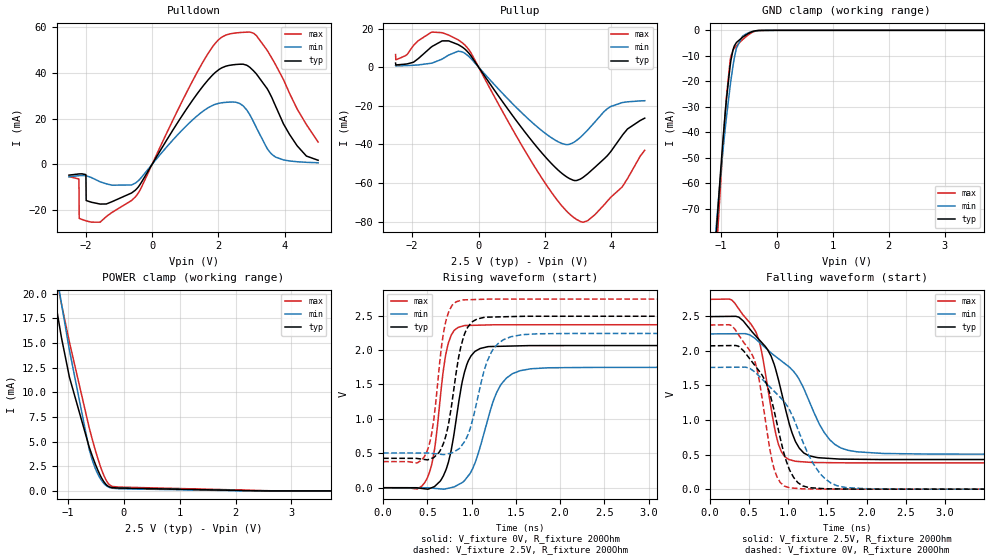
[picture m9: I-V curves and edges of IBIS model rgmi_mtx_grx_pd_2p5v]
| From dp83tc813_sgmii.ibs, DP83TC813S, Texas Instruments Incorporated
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| rgmi_mtx_grx_pd_2p5v
[Model]   rgmi_mtx_grx_pd_2p5v
Model_type   I/O
Polarity   Non-Inverting
Enable   Active-Low
Vinl = 0.7
Vinh = 1.7
Vmeas = 1.25
Vref = 1.25
Cref = 2pF
Rref = 100000
|   typ   min   max
C_comp   1.78pF   1.74pF   1.8pF
[Voltage Range]   2.5   2.25   2.75
[Temperature Range]   27   150   -40
[Pullup Reference]   2.5   2.25   2.75
[Pulldown Reference]   0   0   0
[Power Clamp Reference]   2.5   2.25   2.75
[GND Clamp Reference]   0   0   0
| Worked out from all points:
|   slope of the pulldown table from 0 to 0.375 V, typ, clamps not added: 41.3 ohm
|   slope of the pullup table from 0 to 0.375 V, typ, clamps not added: 39.8 ohm
|   GND clamp passes 1 mA (typ) near -0.49 V on its own axis
|   POWER clamp passes 1 mA (typ) near -0.36 V on its own axis
|   falling waveform, V_fixture 2.5V, R_fixture 200Ohm: 20-80 % time 347ps typ, 578ps min, 245ps max; typ from 2.49 V to 0.427 V
|   rising waveform, V_fixture 0V, R_fixture 200Ohm: 20-80 % time 169ps typ, 257ps min, 133ps max; typ from 0 V to 2.07 V
|   rising waveform, V_fixture 2.5V, R_fixture 200Ohm: 20-80 % time 160ps typ, 215ps min, 129ps max; typ from 0.427 V to 2.49 V
|   falling waveform, V_fixture 0V, R_fixture 200Ohm: 20-80 % time 311ps typ, 501ps min, 225ps max; typ from 2.07 V to 0 V
[Pulldown]
|   Voltage   I(typ)   I(min)   I(max)
-2.5V     -4.672mA   -5.389mA   -5.307mA
-2.208V   -4.173mA   -4.935mA   -6.345mA
-2.2V     -4.164mA   -4.928mA   -6.817mA
-2.192V   -4.156mA   -4.921mA   -23.54mA
-2.118V   -4.109mA   -4.872mA   -23.98mA
-1.99V    -4.622mA   -4.94mA    -24.62mA
-1.982V   -15.77mA   -4.953mA   -24.65mA
-617.5mV  -12.48mA   -8.98mA    -15.76mA
1.587V    35.18mA    23.8mA     46.1mA
2.428V    43.51mA    27.27mA    57.25mA
3.147V    39.41mA    15.86mA    56.18mA
5V        1.822mA    727.1uA    9.773mA
[GND Clamp]
|   Voltage   I(typ)   I(min)   I(max)
-2.5V     -599.2mA   -518.7mA   -673.8mA
-1.097V   -84.65mA   -80.59mA   -94.55mA
-1.045V   -67.67mA   -66.8mA    -74.76mA
-925mV    -32.91mA   -39.02mA   -33.16mA
-902.5mV  -27.45mA   -34.46mA   -26.56mA
-835mV    -13.97mA   -21.96mA   -11.93mA
-782.5mV  -7.567mA   -13.77mA   -7.699mA
-722.5mV  -4.782mA   -7.003mA   -6.022mA
-617.5mV  -2.807mA   -2.423mA   -3.769mA
-520mV    -1.387mA   -1.103mA   -1.953mA
-287.5mV  -43.21uA   -49.05uA   -52.55uA
5V        0A         0A         0A
[Pullup]
|   Voltage   I(typ)   I(min)   I(max)
-2.5V     2.111mA    768.5uA    6.54mA
-2.2V     1.575mA    804.7uA    5.936mA
-1.96V    2.572mA    997.9uA    11.28mA
-1.39V    10.84mA    2.186mA    18.18mA
-902.5mV  13.62mA    6.256mA    16.65mA
-467.5mV  10.11mA    7.704mA    12.3mA
2.083V    -47.91mA   -35.26mA   -62.11mA
2.638V    -56.7mA    -40.12mA   -74.4mA
3.065V    -57.97mA   -36.33mA   -79.98mA
3.973V    -43.87mA   -20.44mA   -67.55mA
4.482V    -32.02mA   -17.96mA   -57.74mA
5V        -26.43mA   -17.39mA   -43.06mA
[POWER Clamp]
|   Voltage   I(typ)   I(min)   I(max)
-2.5V     127.6mA    94.09mA    171.5mA
-1.232V   19.61mA    23.09mA    22.45mA
-1.113V   15.56mA    19mA       18.96mA
-970mV    11.54mA    14.28mA    15.09mA
-617.5mV  4.476mA    4.246mA    6.44mA
-550mV    3.38mA     2.956mA    5.003mA
-460mV    2.088mA    1.696mA    3.259mA
-355mV    942.8uA    770.4uA    1.589mA
-272.5mV  461.3uA    397.3uA    740.3uA
-197.5mV  326.8uA    269.2uA    451.3uA
-25mV     285.4uA    216.3uA    382.5uA
5V        0A         0A         0A
[Ramp]
R_load = 200
|   typ   min   max
dV/dt_r   1.24108/1.68325e-10   1.05398/2.5536e-10   1.42125/1.32406e-10
dV/dt_f   1.23796/3.45009e-10   1.04176/5.77786e-10   1.41626/2.44193e-10
[Falling Waveform]
V_fixture = 2.5V
V_fixture_min = 2.25V
V_fixture_max = 2.75V
R_fixture = 200Ohm
C_fixture = 0F
|   Time   V(typ)   V(min)   V(max)
0s        2.491V     2.241V     2.74V
280.5ps   2.494V     2.243V     2.731V
578.4ps   2.223V     2.176V     2.291V
660.5ps   2.121V     2.092V     1.991V
873.9ps   1.591V     1.886V     658.7mV
1.083ns   716.5mV    1.681V     405.7mV
1.201ns   521.6mV    1.45V      393.8mV
1.529ns   443.4mV    715.6mV    382.4mV
1.881ns   431.5mV    539mV      379.9mV
12ns      427.3mV    504.7mV    379.4mV
[Rising Waveform]
V_fixture = 0V
V_fixture_min = 0V
V_fixture_max = 0V
R_fixture = 200Ohm
C_fixture = 0F
|   Time   V(typ)   V(min)   V(max)
0s        474.9nV    7.945uV    226.6nV
491ps     -18.71mV   -375.4uV   120.6mV
582.9ps   19.67mV    -9.311mV   572.1mV
674.8ps   157.9mV    -19.87mV   1.645V
730.6ps   340mV      -9.567mV   2.066V
919.7ps   1.678V     103.3mV    2.355V
1.041ns   1.982V     367.5mV    2.359V
1.321ns   2.054V     1.475V     2.367V
1.664ns   2.064V     1.726V     2.367V
12ns      2.068V     1.757V     2.369V
[Rising Waveform]
V_fixture = 2.5V
V_fixture_min = 2.25V
V_fixture_max = 2.75V
R_fixture = 200Ohm
C_fixture = 0F
|   Time   V(typ)   V(min)   V(max)
0s        427.3mV    504.7mV    379.4mV
483.4ps   407.6mV    504.3mV    492.2mV
566.5ps   434.5mV    496.5mV    932.1mV
655.8ps   565.4mV    485.1mV    2.006V
708.6ps   751.8mV    486.5mV    2.415V
894.3ps   2.121V     623.4mV    2.727V
1.002ns   2.403V     941.5mV    2.732V
1.224ns   2.479V     1.969V     2.74V
1.567ns   2.489V     2.222V     2.74V
12ns      2.491V     2.241V     2.74V
[Falling Waveform]
|Gnd
V_fixture = 0V
V_fixture_min = 0V
V_fixture_max = 0V
R_fixture = 200Ohm
C_fixture = 0F
|   Time   V(typ)   V(min)   V(max)
0s        2.069V     1.757V     2.369V
279.4ps   2.073V     1.76V      2.361V
544.9ps   1.831V     1.717V     1.932V
626.9ps   1.711V     1.635V     1.598V
815.3ps   1.165V     1.421V     318mV
1.018ns   282.2mV    1.145V     20.22mV
1.186ns   47.1mV     688.3mV    4.798mV
1.394ns   12.08mV    245.4mV    1.121mV
1.738ns   2.289mV    23.36mV    177.9uV
12ns      632.3nV    8.21uV     319.6nV
